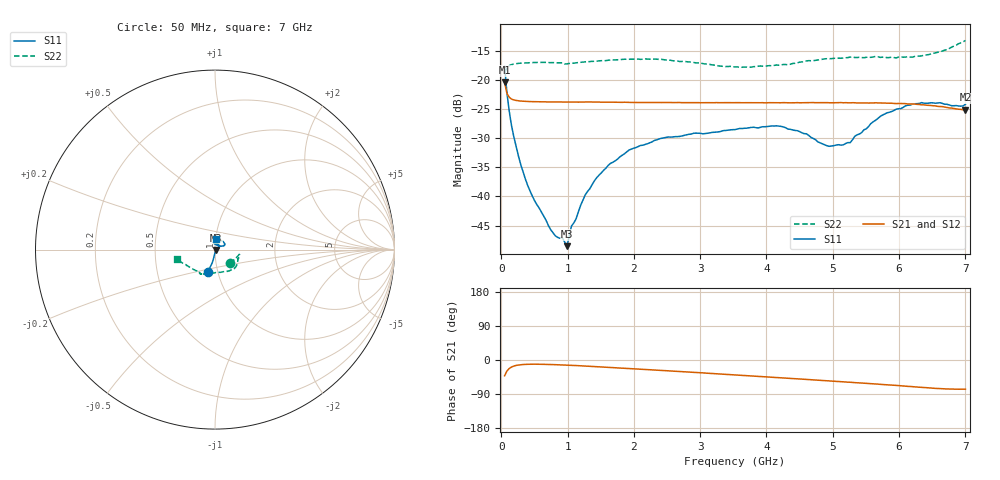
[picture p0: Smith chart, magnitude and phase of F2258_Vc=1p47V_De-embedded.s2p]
! Integrated Device Technology
! Corporate Headquarters
! 6024 Silver Creek Valley Road
! San Jose, CA 95138  USA
! Phone:  1-408-284-8200
! Toll Free:  1-800-223-1366
! Webpage:  http://www.idt.com/
! Timing and RF Division
! 515 Groton Road, Suite 102
! Westford, MA 01886-6024
! Device:  F2258
! Description: Voltage Variable RF Attenuator
! Frequency:  50.0 -  6000.00 MHz
! Package:  3x3 mm Thin QFN Plastic Package: 16 pin
! Ports:  2 RF, 2 DC
!  Pin  1  = NC
!  Pin  2  = NC
!  Pin  3  = RF2  = Port 2
!  Pin  4  = GND
!  Pin  5  = Vdd
!  Pin  6  = NC
!  Pin  7  = VCTRL
!  Pin  8  = NC
!  Pin  9  = GND
!  Pin 10  = RF1  = Port 1
!  Pin 11  = NC
!  Pin 12  = NC
!  Pin 13  = NC
!  Pin 14  = NC
!  Pin 15  = NC
!  Pin 16  = NC
! Vcntrl:  1.470 Volts
! Vdd:  +3.300 Volts
! Current:  1.165 mA
! Data:  The device was measured on a the F2258 evaluation board which has
!  individual transmission lines to the RF pins.  Data was collected
!  using a calibrated network analyzer.  The evaluation board was
!  de-embedded using a TRL calibration technique.
!  The reference plane is the edge of the package pin.
! Misc:  SN 10
!  Action Tracker AT0285
! Date Measured:  2014-12-10
! Date:  2016-01-13  MJV
! Note:
!  Integrated Device Technology supplies this data as a sample of measured
!  data at the package pin for this product.  Your particular data for this
!  product may vary.
!  Data was taken at 25 degrees C.
!  Integrated Device Technology reserves the right to change this data at anytime.
!Freq_(GHz)  S11M_(dB)  S11P_(deg)  S21M_(dB)  S21P_(deg)  S12M_(dB)  S12P_(deg)  S22M_(dB)  S22P_(deg)
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# GHz S dB R 50
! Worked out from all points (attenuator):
!   201 points, 50 MHz to 7 GHz, reference 50 ohm
!   highest |S21| = -20.42 dB at 50 MHz (marker M1); lowest = -25.1 dB at 7 GHz (marker M2)
!   lowest |S11| = -48.5 dB at 988.2 MHz (marker M3), VSWR 1.01, Z = 50.3 - j0.233 ohm
!   |S11| at or under -10 dB: start of sweep to end of sweep
!   |S22| runs from -18.9 to -13.3 dB; largest |S21 - S12| = 0.0003
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0.05  -17.70 -107.6  -20.42 -41.6  -20.42 -41.6  -18.86 -42.4
0.08475  -22.17 -102.3  -22.33 -29.2  -22.32 -29.2  -17.96 -21.8
0.15425  -27.85 -98.4  -23.30 -18.5  -23.28 -18.5  -17.39 -13.4
0.2585  -33.06 -94.5  -23.60 -13.2  -23.60 -13.2  -17.18 -10.9
0.36275  -36.99 -90.4  -23.69 -11.5  -23.68 -11.5  -17.10 -11.4
0.745  -45.70 -52.5  -23.78 -11.9  -23.80 -11.9  -17.07 -17.2
0.91875  -46.97 -7.3  -23.80 -13.1  -23.84 -13.1  -17.08 -21.0
0.98825  -48.52 -38.1  -23.81 -13.6  -23.82 -13.6  -17.27 -22.1
1.05775  -45.10 -15.7  -23.82 -14.1  -23.84 -14.1  -17.15 -23.3
1.2315  -40.62 4.5  -23.81 -15.6  -23.81 -15.6  -16.95 -26.5
1.44  -36.77 10.2  -23.82 -17.7  -23.83 -17.7  -16.81 -30.3
1.6485  -34.32 15.1  -23.83 -19.8  -23.85 -19.8  -16.62 -33.9
1.9265  -32.05 24.2  -23.89 -22.6  -23.88 -22.6  -16.48 -38.6
2.37825  -30.14 35.8  -23.92 -27.1  -23.90 -27.1  -16.50 -46.7
3.525  -28.54 85.8  -23.92 -39.4  -23.92 -39.4  -17.80 -79.1
4.1505  -27.89 102.8  -23.92 -46.3  -23.95 -46.2  -17.46 -101.3
4.7065  -30.06 92.8  -23.90 -52.4  -23.93 -52.4  -16.72 -113.2
4.94975  -31.41 74.6  -23.94 -55.1  -23.95 -55.1  -16.38 -115.7
5.2625  -30.78 45.2  -23.96 -58.7  -23.98 -58.7  -16.11 -118.2
5.85325  -25.57 24.0  -24.01 -66.0  -24.02 -66.0  -16.18 -123.7
6.33975  -23.91 30.8  -24.29 -72.3  -24.30 -72.3  -15.90 -135.7
7  -24.20 83.5  -25.14 -76.9  -25.14 -76.9  -13.25 -165.3
